FUNCTION "SEGNALAZIONI" : VOID
TITLE =SEGNALAZIONI
VERSION : 0.1

BEGIN
NETWORK
TITLE =SEGN 1 = TEMPERATURA MIN FORNO
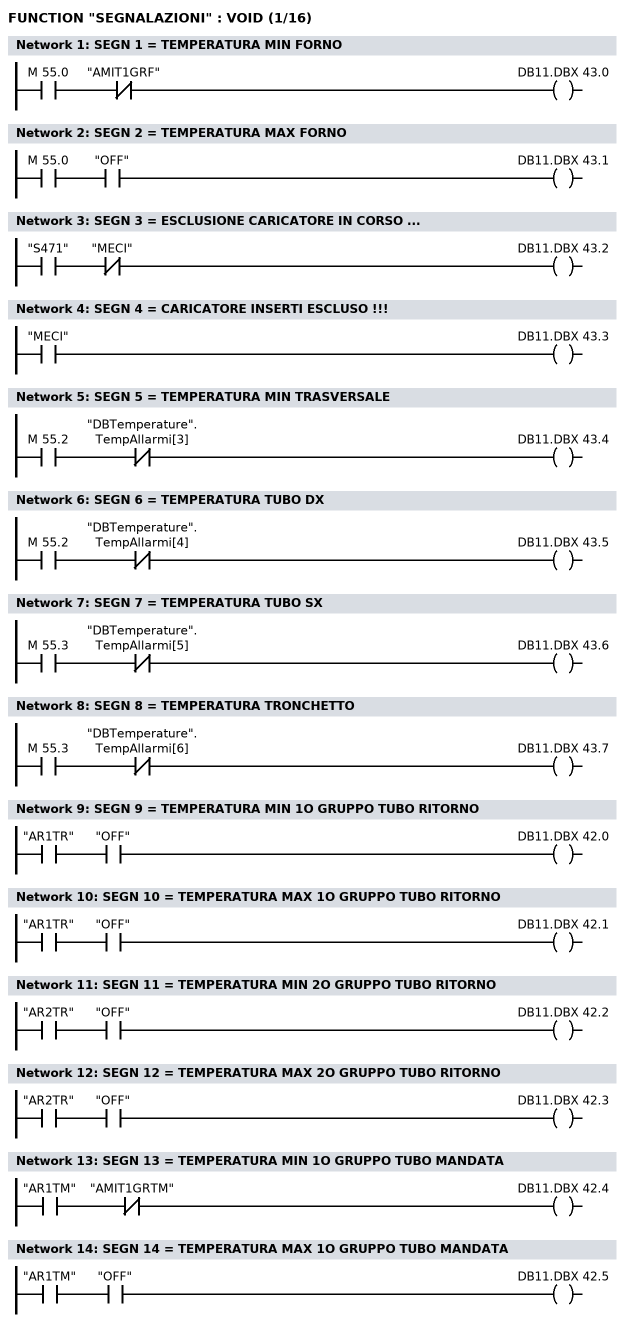
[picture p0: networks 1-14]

      U     M     55.0;
      UN    "AMIT1GRF";
      =     DB11.DBX   43.0;
NETWORK
TITLE =SEGN 2 = TEMPERATURA MAX FORNO

      U     M     55.0;
      U     "OFF";
      =     DB11.DBX   43.1;
NETWORK
TITLE =SEGN 3 = ESCLUSIONE CARICATORE IN CORSO ...

      U     "S471";
      UN    "MECI";
      =     DB11.DBX   43.2;
NETWORK
TITLE =SEGN 4 = CARICATORE INSERTI ESCLUSO !!!

      U     "MECI";
      =     DB11.DBX   43.3;
NETWORK
TITLE =SEGN 5 = TEMPERATURA MIN TRASVERSALE

      U     M     55.2;
      UN    "DBTemperature".TempAllarmi[3];
      =     DB11.DBX   43.4;
NETWORK
TITLE =SEGN 6 = TEMPERATURA TUBO DX

      U     M     55.2;
      UN    "DBTemperature".TempAllarmi[4];
      =     DB11.DBX   43.5;
NETWORK
TITLE =SEGN 7 = TEMPERATURA TUBO SX

      U     M     55.3;
      UN    "DBTemperature".TempAllarmi[5];
      =     DB11.DBX   43.6;
NETWORK
TITLE =SEGN 8 = TEMPERATURA TRONCHETTO

      U     M     55.3;
      UN    "DBTemperature".TempAllarmi[6];
      =     DB11.DBX   43.7;
NETWORK
TITLE =SEGN 9 = TEMPERATURA MIN 1O GRUPPO TUBO RITORNO

      U     "AR1TR";
      U     "OFF";
      =     DB11.DBX   42.0;
NETWORK
TITLE =SEGN 10 = TEMPERATURA MAX 1O GRUPPO TUBO RITORNO

      U     "AR1TR";
      U     "OFF";
      =     DB11.DBX   42.1;
NETWORK
TITLE =SEGN 11 = TEMPERATURA MIN 2O GRUPPO TUBO RITORNO

      U     "AR2TR";
      U     "OFF";
      =     DB11.DBX   42.2;
NETWORK
TITLE =SEGN 12 = TEMPERATURA MAX 2O GRUPPO TUBO RITORNO

      U     "AR2TR";
      U     "OFF";
      =     DB11.DBX   42.3;
NETWORK
TITLE =SEGN 13 = TEMPERATURA MIN 1O GRUPPO TUBO MANDATA

      U     "AR1TM";
      UN    "AMIT1GRTM";
      =     DB11.DBX   42.4;
NETWORK
TITLE =SEGN 14 = TEMPERATURA MAX 1O GRUPPO TUBO MANDATA

      U     "AR1TM";
      U     "OFF";
      =     DB11.DBX   42.5;
NETWORK
TITLE =SEGN 15 = TEMPERATURA MIN 2O GRUPPO TUBO MANDATA
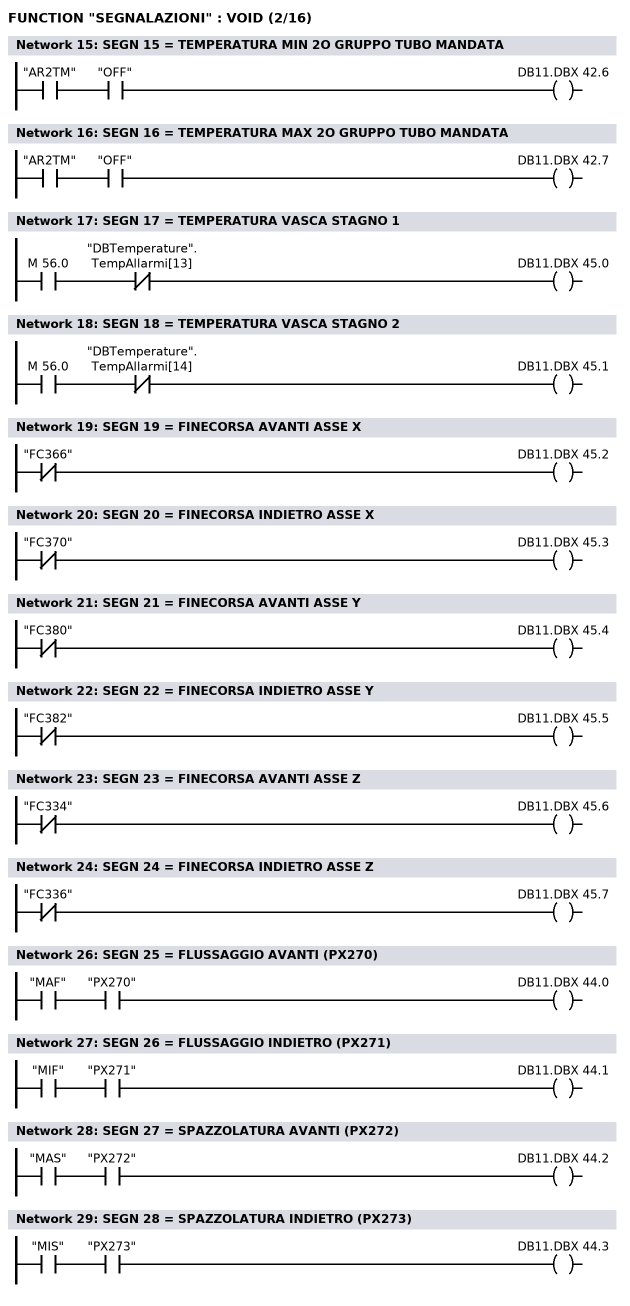
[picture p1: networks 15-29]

      U     "AR2TM";
      U     "OFF";
      =     DB11.DBX   42.6;
NETWORK
TITLE =SEGN 16 = TEMPERATURA MAX 2O GRUPPO TUBO MANDATA

      U     "AR2TM";
      U     "OFF";
      =     DB11.DBX   42.7;
NETWORK
TITLE =SEGN 17 = TEMPERATURA VASCA STAGNO 1

      U     M     56.0;
      UN    "DBTemperature".TempAllarmi[13];
      =     DB11.DBX   45.0;
NETWORK
TITLE =SEGN 18 = TEMPERATURA VASCA STAGNO 2

      U     M     56.0;
      UN    "DBTemperature".TempAllarmi[14];
      =     DB11.DBX   45.1;
NETWORK
TITLE =SEGN 19 = FINECORSA AVANTI ASSE X

      UN    "FC366";
      =     DB11.DBX   45.2;
NETWORK
TITLE =SEGN 20 = FINECORSA INDIETRO ASSE X

      UN    "FC370";
      =     DB11.DBX   45.3;
NETWORK
TITLE =SEGN 21 = FINECORSA AVANTI ASSE Y

      UN    "FC380";
      =     DB11.DBX   45.4;
NETWORK
TITLE =SEGN 22 = FINECORSA INDIETRO ASSE Y

      UN    "FC382";
      =     DB11.DBX   45.5;
NETWORK
TITLE =SEGN 23 = FINECORSA AVANTI ASSE Z

      UN    "FC334";
      =     DB11.DBX   45.6;
NETWORK
TITLE =SEGN 24 = FINECORSA INDIETRO ASSE Z

      UN    "FC336";
      =     DB11.DBX   45.7;
NETWORK
TITLE =

// ###########################################
// CONDIZIONI MOVIMENTI MANUALI
// ###########################################
NETWORK
TITLE =SEGN 25 = FLUSSAGGIO AVANTI (PX270)

      U     "MAF";
      U     "PX270";
      =     DB11.DBX   44.0;
NETWORK
TITLE =SEGN 26 = FLUSSAGGIO INDIETRO (PX271)

      U     "MIF";
      U     "PX271";
      =     DB11.DBX   44.1;
NETWORK
TITLE =SEGN 27 = SPAZZOLATURA AVANTI (PX272)

      U     "MAS";
      U     "PX272";
      =     DB11.DBX   44.2;
NETWORK
TITLE =SEGN 28 = SPAZZOLATURA INDIETRO (PX273)

      U     "MIS";
      U     "PX273";
      =     DB11.DBX   44.3;
NETWORK
TITLE =BIT TEST CONDIZIONI START ROTAZIONE
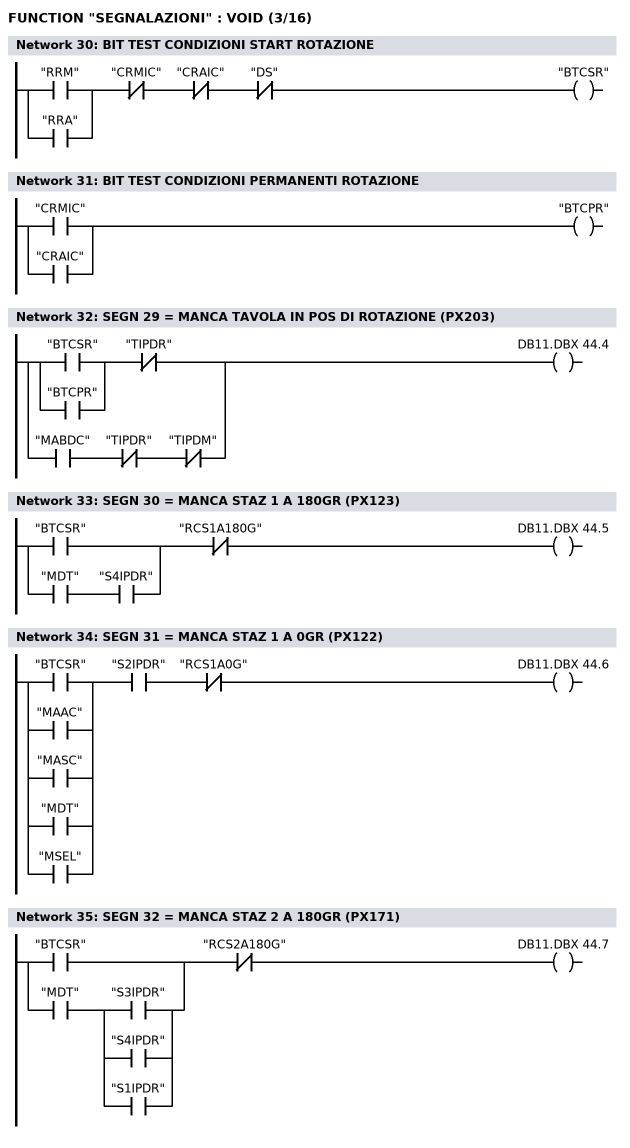
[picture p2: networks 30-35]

      U(    ;
      O     "RRM";
      O     "RRA";
      )     ;
      UN    "CRMIC";
      UN    "CRAIC";
      UN    "DS";
      =     "BTCSR";
NETWORK
TITLE =BIT TEST CONDIZIONI PERMANENTI ROTAZIONE

      O     "CRMIC";
      O     "CRAIC";
      =     "BTCPR";
NETWORK
TITLE =SEGN 29 = MANCA TAVOLA IN POS DI ROTAZIONE (PX203)

      U(    ;
      O     "BTCSR";
      O     "BTCPR";
      )     ;
      UN    "TIPDR";
      O     ;
      U     "MABDC";
      UN    "TIPDR";
      UN    "TIPDM";
      =     DB11.DBX   44.4;
NETWORK
TITLE =SEGN 30 = MANCA STAZ 1 A 180GR (PX123)

      U(    ;
      O     "BTCSR";
      O     ;
      U     "MDT";
      U     "S4IPDR";
      )     ;
      UN    "RCS1A180G";
      =     DB11.DBX   44.5;
NETWORK
TITLE =SEGN 31 = MANCA STAZ 1 A 0GR (PX122)

      U(    ;
      O     "BTCSR";
      O     "MAAC";
      O     "MASC";
      O     "MDT";
      O     "MSEL";
      )     ;
      U     "S2IPDR";
      UN    "RCS1A0G";
      =     DB11.DBX   44.6;
NETWORK
TITLE =SEGN 32 = MANCA STAZ 2 A 180GR (PX171)

      U(    ;
      O     "BTCSR";
      O     ;
      U     "MDT";
      U(    ;
      O     "S3IPDR";
      O     "S4IPDR";
      O     "S1IPDR";
      )     ;
      )     ;
      UN    "RCS2A180G";
      =     DB11.DBX   44.7;
NETWORK
TITLE =SEGN 33 = MANCA STAZ 2 A 0GR (PX170)
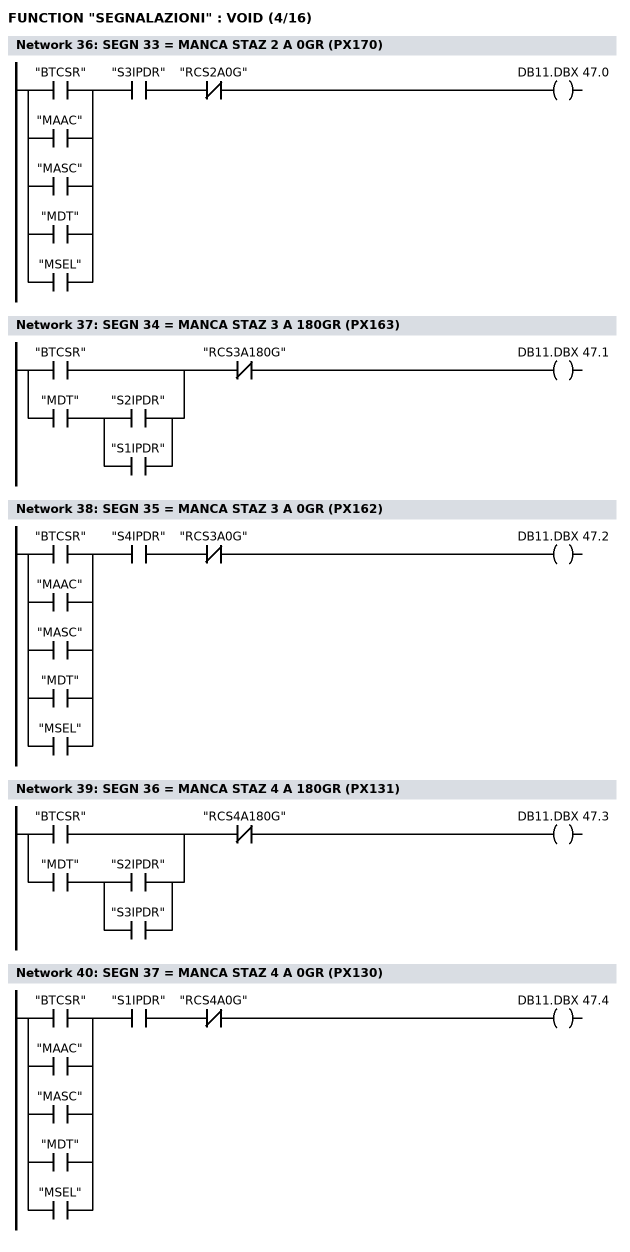
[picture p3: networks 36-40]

      U(    ;
      O     "BTCSR";
      O     "MAAC";
      O     "MASC";
      O     "MDT";
      O     "MSEL";
      )     ;
      U     "S3IPDR";
      UN    "RCS2A0G";
      =     DB11.DBX   47.0;
NETWORK
TITLE =SEGN 34 = MANCA STAZ 3 A 180GR (PX163)

      U(    ;
      O     "BTCSR";
      O     ;
      U     "MDT";
      U(    ;
      O     "S2IPDR";
      O     "S1IPDR";
      )     ;
      )     ;
      UN    "RCS3A180G";
      =     DB11.DBX   47.1;
NETWORK
TITLE =SEGN 35 = MANCA STAZ 3 A 0GR (PX162)

      U(    ;
      O     "BTCSR";
      O     "MAAC";
      O     "MASC";
      O     "MDT";
      O     "MSEL";
      )     ;
      U     "S4IPDR";
      UN    "RCS3A0G";
      =     DB11.DBX   47.2;
NETWORK
TITLE =SEGN 36 = MANCA STAZ 4 A 180GR (PX131)

      U(    ;
      O     "BTCSR";
      O     ;
      U     "MDT";
      U(    ;
      O     "S2IPDR";
      O     "S3IPDR";
      )     ;
      )     ;
      UN    "RCS4A180G";
      =     DB11.DBX   47.3;
NETWORK
TITLE =SEGN 37 = MANCA STAZ 4 A 0GR (PX130)

      U(    ;
      O     "BTCSR";
      O     "MAAC";
      O     "MASC";
      O     "MDT";
      O     "MSEL";
      )     ;
      U     "S1IPDR";
      UN    "RCS4A0G";
      =     DB11.DBX   47.4;
NETWORK
TITLE =SEGN 38 = MANCA BRACCIO DI CARICO INDIETRO (QUOTA)
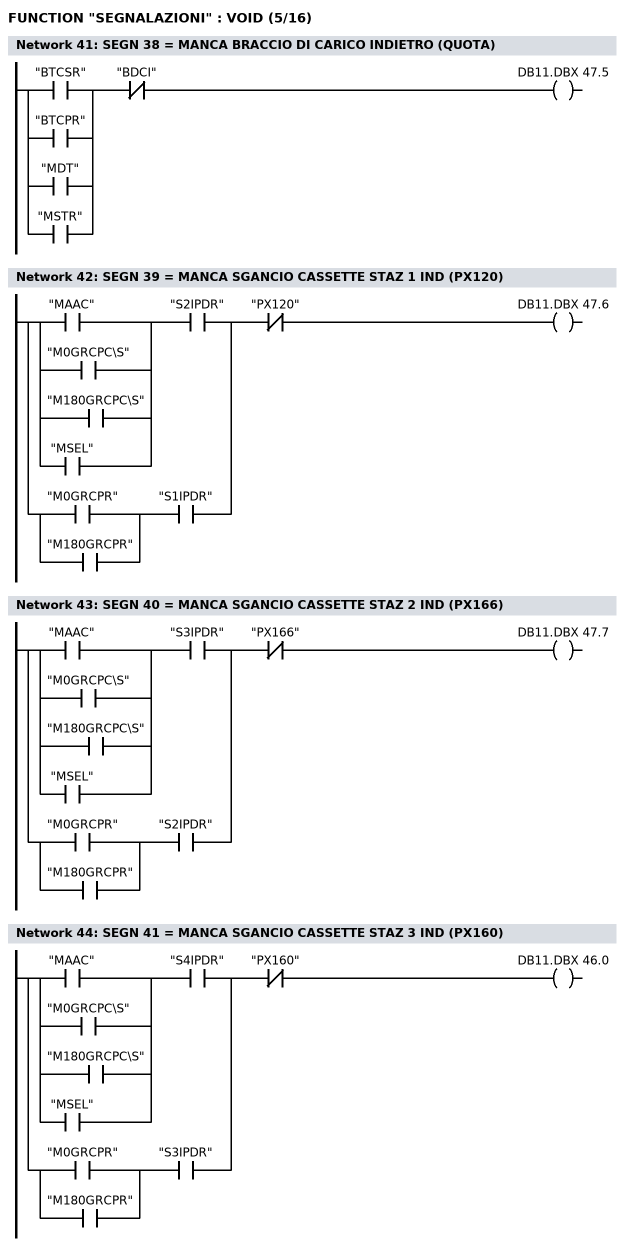
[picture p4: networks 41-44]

      U(    ;
      O     "BTCSR";
      O     "BTCPR";
      O     "MDT";
      O     "MSTR";
      )     ;
      UN    "BDCI";
      =     DB11.DBX   47.5;
NETWORK
TITLE =SEGN 39 = MANCA SGANCIO CASSETTE STAZ 1 IND (PX120)

      U(    ;
      U(    ;
      O     "MAAC";
      O     "M0GRCPC\S";
      O     "M180GRCPC\S";
      O     "MSEL";
      )     ;
      U     "S2IPDR";
      O     ;
      U(    ;
      O     "M0GRCPR";
      O     "M180GRCPR";
      )     ;
      U     "S1IPDR";
      )     ;
      UN    "PX120";
      =     DB11.DBX   47.6;
NETWORK
TITLE =SEGN 40 = MANCA SGANCIO CASSETTE STAZ 2 IND (PX166)

      U(    ;
      U(    ;
      O     "MAAC";
      O     "M0GRCPC\S";
      O     "M180GRCPC\S";
      O     "MSEL";
      )     ;
      U     "S3IPDR";
      O     ;
      U(    ;
      O     "M0GRCPR";
      O     "M180GRCPR";
      )     ;
      U     "S2IPDR";
      )     ;
      UN    "PX166";
      =     DB11.DBX   47.7;
NETWORK
TITLE =SEGN 41 = MANCA SGANCIO CASSETTE STAZ 3 IND (PX160)

      U(    ;
      U(    ;
      O     "MAAC";
      O     "M0GRCPC\S";
      O     "M180GRCPC\S";
      O     "MSEL";
      )     ;
      U     "S4IPDR";
      O     ;
      U(    ;
      O     "M0GRCPR";
      O     "M180GRCPR";
      )     ;
      U     "S3IPDR";
      )     ;
      UN    "PX160";
      =     DB11.DBX   46.0;
NETWORK
TITLE =SEGN 42 = MANCA SGANCIO CASSETTE STAZ 4 IND (PX126)
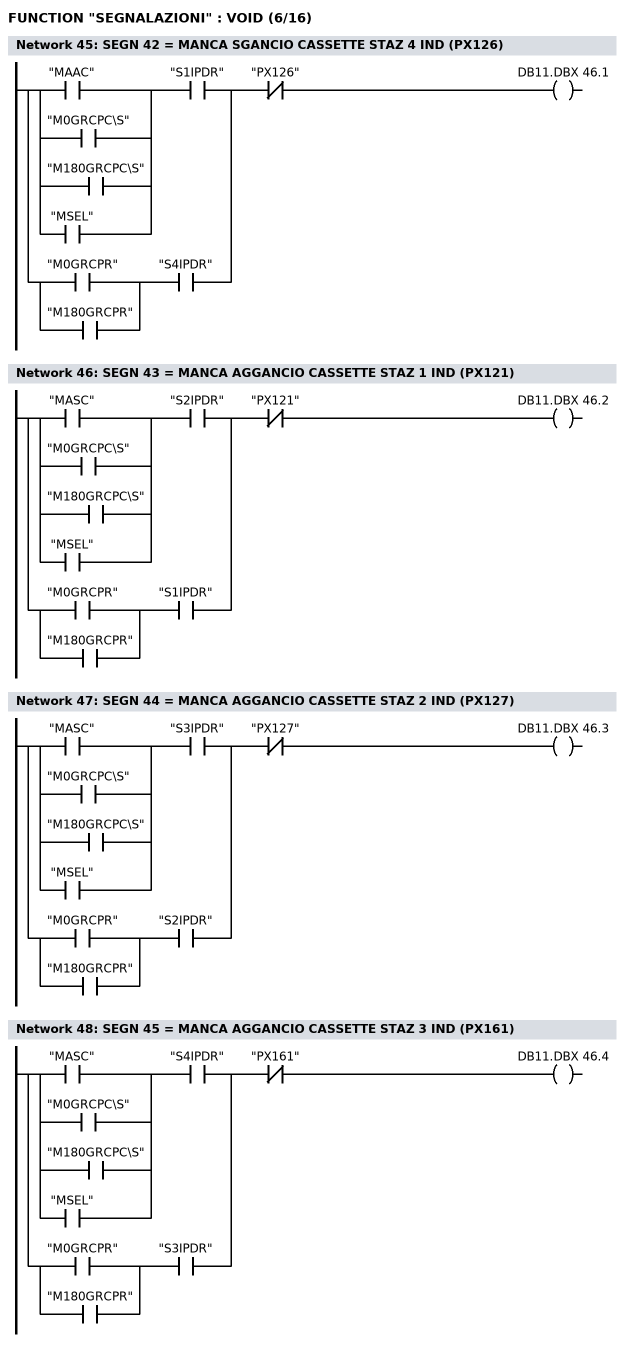
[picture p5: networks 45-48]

      U(    ;
      U(    ;
      O     "MAAC";
      O     "M0GRCPC\S";
      O     "M180GRCPC\S";
      O     "MSEL";
      )     ;
      U     "S1IPDR";
      O     ;
      U(    ;
      O     "M0GRCPR";
      O     "M180GRCPR";
      )     ;
      U     "S4IPDR";
      )     ;
      UN    "PX126";
      =     DB11.DBX   46.1;
NETWORK
TITLE =SEGN 43 = MANCA AGGANCIO CASSETTE STAZ 1 IND (PX121)

      U(    ;
      U(    ;
      O     "MASC";
      O     "M0GRCPC\S";
      O     "M180GRCPC\S";
      O     "MSEL";
      )     ;
      U     "S2IPDR";
      O     ;
      U(    ;
      O     "M0GRCPR";
      O     "M180GRCPR";
      )     ;
      U     "S1IPDR";
      )     ;
      UN    "PX121";
      =     DB11.DBX   46.2;
NETWORK
TITLE =SEGN 44 = MANCA AGGANCIO CASSETTE STAZ 2 IND (PX127)

      U(    ;
      U(    ;
      O     "MASC";
      O     "M0GRCPC\S";
      O     "M180GRCPC\S";
      O     "MSEL";
      )     ;
      U     "S3IPDR";
      O     ;
      U(    ;
      O     "M0GRCPR";
      O     "M180GRCPR";
      )     ;
      U     "S2IPDR";
      )     ;
      UN    "PX127";
      =     DB11.DBX   46.3;
NETWORK
TITLE =SEGN 45 = MANCA AGGANCIO CASSETTE STAZ 3 IND (PX161)

      U(    ;
      U(    ;
      O     "MASC";
      O     "M0GRCPC\S";
      O     "M180GRCPC\S";
      O     "MSEL";
      )     ;
      U     "S4IPDR";
      O     ;
      U(    ;
      O     "M0GRCPR";
      O     "M180GRCPR";
      )     ;
      U     "S3IPDR";
      )     ;
      UN    "PX161";
      =     DB11.DBX   46.4;
NETWORK
TITLE =SEGN 46 = MANCA AGGANCIO CASSETTE STAZ 4 IND (PX167)
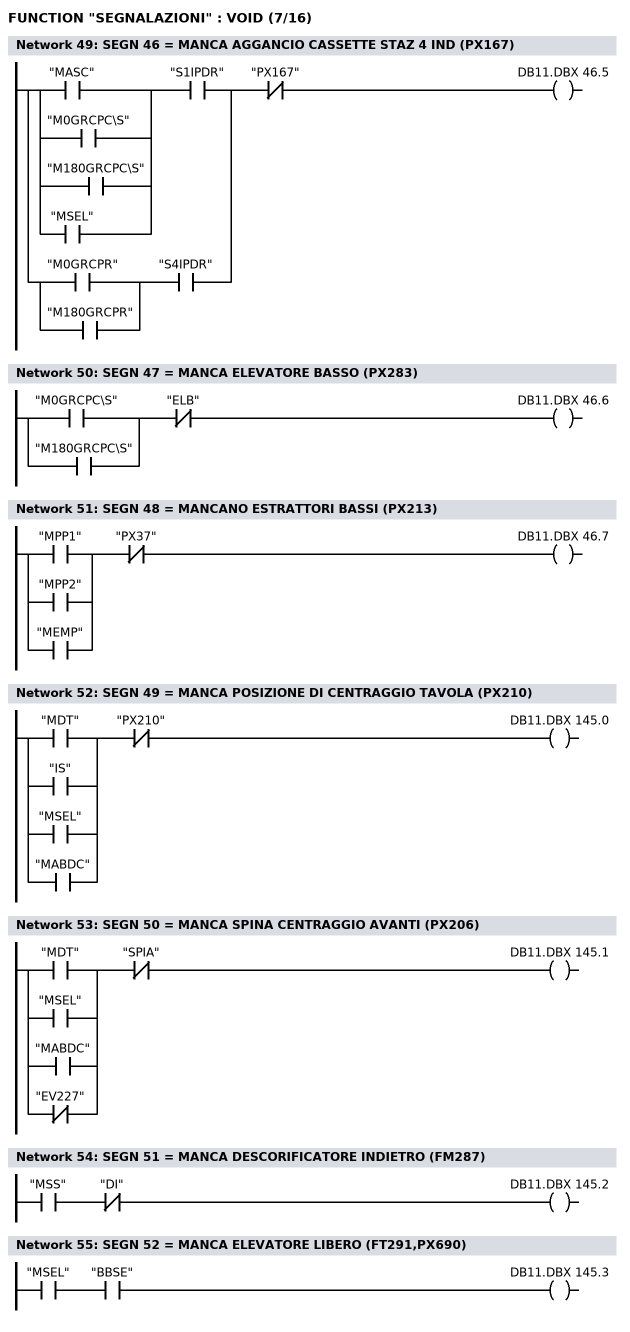
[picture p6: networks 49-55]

      U(    ;
      U(    ;
      O     "MASC";
      O     "M0GRCPC\S";
      O     "M180GRCPC\S";
      O     "MSEL";
      )     ;
      U     "S1IPDR";
      O     ;
      U(    ;
      O     "M0GRCPR";
      O     "M180GRCPR";
      )     ;
      U     "S4IPDR";
      )     ;
      UN    "PX167";
      =     DB11.DBX   46.5;
NETWORK
TITLE =SEGN 47 = MANCA ELEVATORE BASSO (PX283)

      U(    ;
      O     "M0GRCPC\S";
      O     "M180GRCPC\S";
      )     ;
      UN    "ELB";
      =     DB11.DBX   46.6;
NETWORK
TITLE =SEGN 48 = MANCANO ESTRATTORI BASSI (PX213)

      U(    ;
      O     "MPP1";
      O     "MPP2";
      O     "MEMP";
      )     ;
      UN    "PX37";
      =     DB11.DBX   46.7;
NETWORK
TITLE =SEGN 49 = MANCA POSIZIONE DI CENTRAGGIO TAVOLA (PX210)

      U(    ;
      O     "MDT";
      O     "IS";
      O     "MSEL";
      O     "MABDC";
      )     ;
      UN    "PX210";
      =     DB11.DBX  145.0;
NETWORK
TITLE =SEGN 50 = MANCA SPINA CENTRAGGIO AVANTI (PX206)

      U(    ;
      O     "MDT";
      O     "MSEL";
      O     "MABDC";
      ON    "EV227";
      )     ;
      UN    "SPIA";
      =     DB11.DBX  145.1;
NETWORK
TITLE =SEGN 51 = MANCA DESCORIFICATORE INDIETRO (FM287)

      U     "MSS";
      UN    "DI";
      =     DB11.DBX  145.2;
NETWORK
TITLE =SEGN 52 = MANCA ELEVATORE LIBERO (FT291,PX690)

      U     "MSEL";
      U     "BBSE";
      =     DB11.DBX  145.3;
NETWORK
TITLE =SEGN 53 = MANCA STAGNATURA BASSA (PX285)
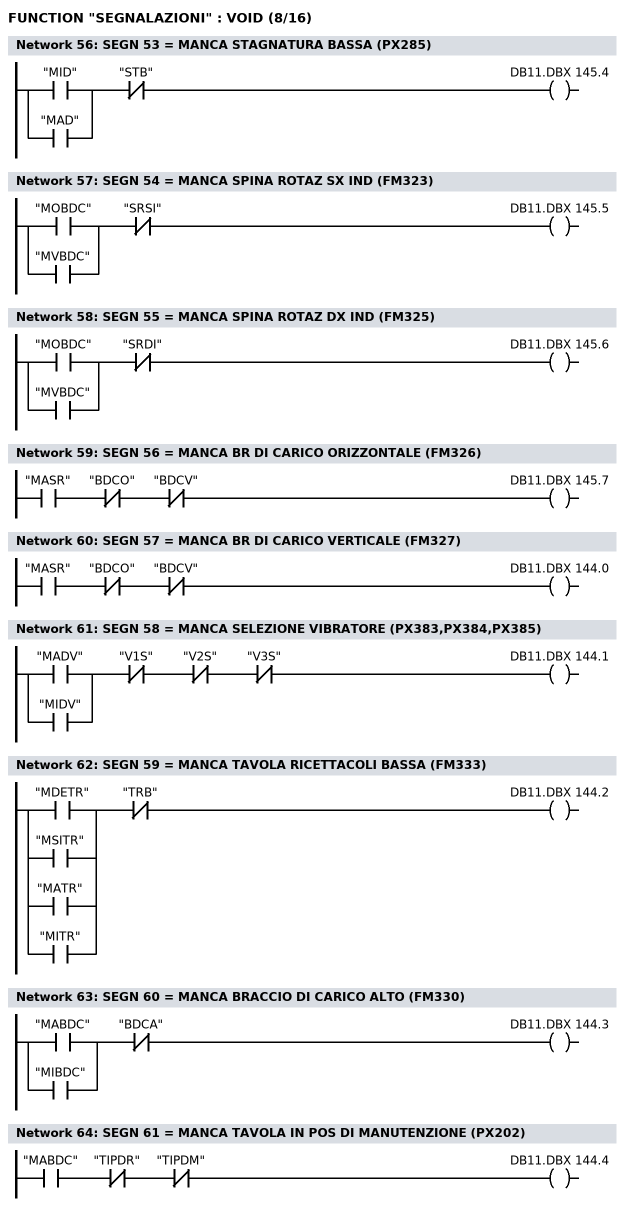
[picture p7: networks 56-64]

      U(    ;
      O     "MID";
      O     "MAD";
      )     ;
      UN    "STB";
      =     DB11.DBX  145.4;
NETWORK
TITLE =SEGN 54 = MANCA SPINA ROTAZ SX IND (FM323)

      U(    ;
      O     "MOBDC";
      O     "MVBDC";
      )     ;
      UN    "SRSI";
      =     DB11.DBX  145.5;
NETWORK
TITLE =SEGN 55 = MANCA SPINA ROTAZ DX IND (FM325)

      U(    ;
      O     "MOBDC";
      O     "MVBDC";
      )     ;
      UN    "SRDI";
      =     DB11.DBX  145.6;
NETWORK
TITLE =SEGN 56 = MANCA BR DI CARICO ORIZZONTALE (FM326)

      U     "MASR";
      UN    "BDCO";
      UN    "BDCV";
      =     DB11.DBX  145.7;
NETWORK
TITLE =SEGN 57 = MANCA BR DI CARICO VERTICALE (FM327)

      U     "MASR";
      UN    "BDCO";
      UN    "BDCV";
      =     DB11.DBX  144.0;
NETWORK
TITLE =SEGN 58 = MANCA SELEZIONE VIBRATORE (PX383,PX384,PX385)

      U(    ;
      O     "MADV";
      O     "MIDV";
      )     ;
      UN    "V1S";
      UN    "V2S";
      UN    "V3S";
      =     DB11.DBX  144.1;
NETWORK
TITLE =SEGN 59 = MANCA TAVOLA RICETTACOLI BASSA (FM333)

      U(    ;
      O     "MDETR";
      O     "MSITR";
      O     "MATR";
      O     "MITR";
      )     ;
      UN    "TRB";
      =     DB11.DBX  144.2;
NETWORK
TITLE =SEGN 60 = MANCA BRACCIO DI CARICO ALTO (FM330)

      U(    ;
      O     "MABDC";
      O     "MIBDC";
      )     ;
      UN    "BDCA";
      =     DB11.DBX  144.3;
NETWORK
TITLE =SEGN 61 = MANCA TAVOLA IN POS DI MANUTENZIONE (PX202)

      U     "MABDC";
      UN    "TIPDR";
      UN    "TIPDM";
      =     DB11.DBX  144.4;
NETWORK
TITLE =SEGN 62 = MANCA POSIZIONE STAZIONI (PX114,PX115,PX116,PX117)
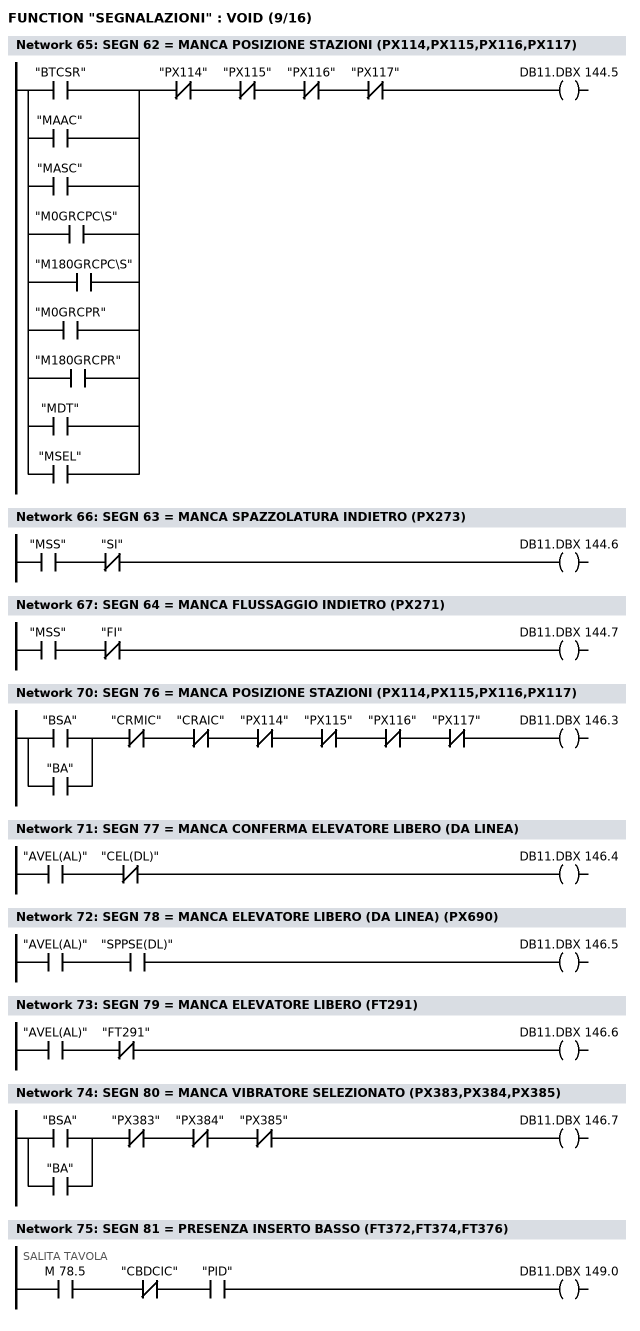
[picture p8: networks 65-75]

      U(    ;
      O     "BTCSR";
      O     "MAAC";
      O     "MASC";
      O     "M0GRCPC\S";
      O     "M180GRCPC\S";
      O     "M0GRCPR";
      O     "M180GRCPR";
      O     "MDT";
      O     "MSEL";
      )     ;
      UN    "PX114";
      UN    "PX115";
      UN    "PX116";
      UN    "PX117";
      =     DB11.DBX  144.5;
NETWORK
TITLE =SEGN 63 = MANCA SPAZZOLATURA INDIETRO (PX273)

      U     "MSS";
      UN    "SI";
      =     DB11.DBX  144.6;
NETWORK
TITLE =SEGN 64 = MANCA FLUSSAGGIO INDIETRO (PX271)

      U     "MSS";
      UN    "FI";
      =     DB11.DBX  144.7;
NETWORK
TITLE =

// SEGN 65-72 DBB147
// SEGN 73-80 DBB146
NETWORK
TITLE =

// ###########################################
// CONTROLLO SEGNALI SENZA COMANDO
// ###########################################
NETWORK
TITLE =SEGN 76 = MANCA POSIZIONE STAZIONI (PX114,PX115,PX116,PX117)

      U(    ;
      O     "BSA";
      O     "BA";
      )     ;
      UN    "CRMIC";
      UN    "CRAIC";
      UN    "PX114";
      UN    "PX115";
      UN    "PX116";
      UN    "PX117";
      =     DB11.DBX  146.3;
NETWORK
TITLE =SEGN 77 = MANCA CONFERMA ELEVATORE LIBERO (DA LINEA)

      U     "AVEL(AL)";
      UN    "CEL(DL)";
      =     DB11.DBX  146.4;
NETWORK
TITLE =SEGN 78 = MANCA ELEVATORE LIBERO (DA LINEA) (PX690)

      U     "AVEL(AL)";
      U     "SPPSE(DL)";
      =     DB11.DBX  146.5;
NETWORK
TITLE =SEGN 79 = MANCA ELEVATORE LIBERO (FT291)

      U     "AVEL(AL)";
      UN    "FT291";
      =     DB11.DBX  146.6;
NETWORK
TITLE =SEGN 80 = MANCA VIBRATORE SELEZIONATO (PX383,PX384,PX385)

      U(    ;
      O     "BSA";
      O     "BA";
      )     ;
      UN    "PX383";
      UN    "PX384";
      UN    "PX385";
      =     DB11.DBX  146.7;
NETWORK
TITLE =SEGN 81 = PRESENZA INSERTO BASSO (FT372,FT374,FT376)

      U     M     78.5; // SALITA TAVOLA
      UN    "CBDCIC";
      U     "PID";
      =     DB11.DBX  149.0;
NETWORK
TITLE =SEGN 82 = MANCA BRACCIO DI CARICO ALTO (FM330)
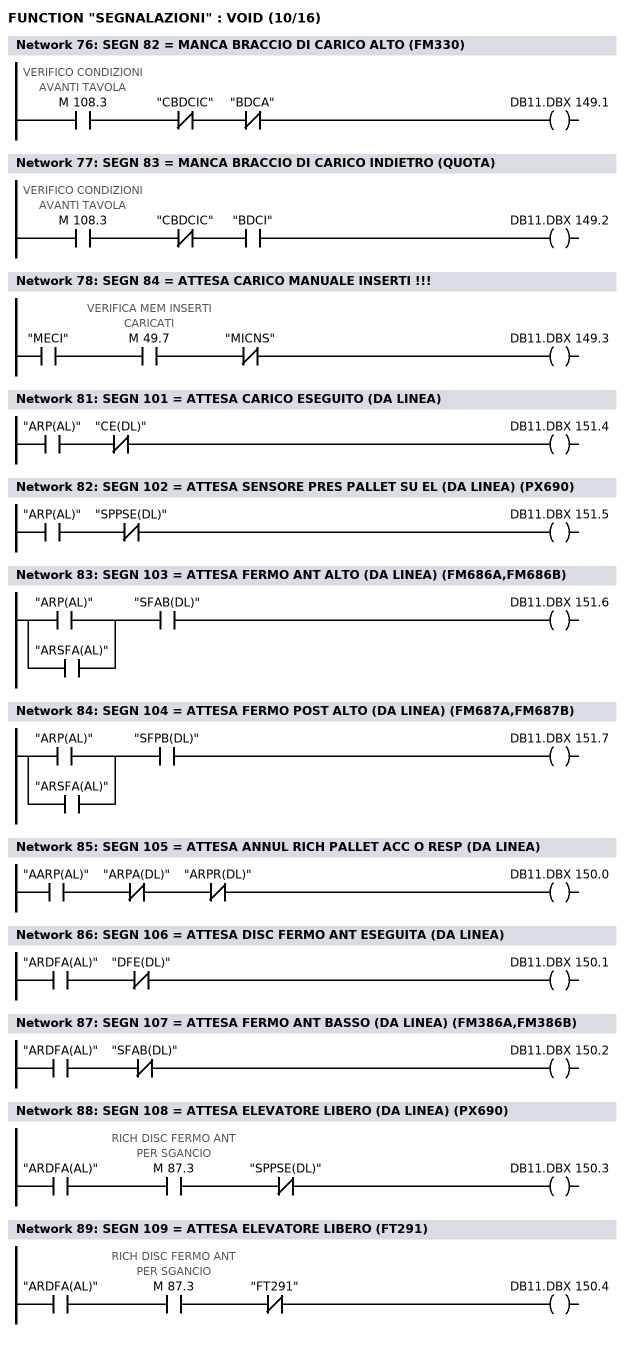
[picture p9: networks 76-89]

      U     M    108.3; // VERIFICO CONDIZIONI AVANTI TAVOLA
      UN    "CBDCIC";
      UN    "BDCA";
      =     DB11.DBX  149.1;
NETWORK
TITLE =SEGN 83 = MANCA BRACCIO DI CARICO INDIETRO (QUOTA)

      U     M    108.3; // VERIFICO CONDIZIONI AVANTI TAVOLA
      UN    "CBDCIC";
      U     "BDCI";
      =     DB11.DBX  149.2;
NETWORK
TITLE =SEGN 84 = ATTESA CARICO MANUALE INSERTI !!!

      U     "MECI";
      U     M     49.7; // VERIFICA MEM INSERTI CARICATI
      UN    "MICNS";
      =     DB11.DBX  149.3;
NETWORK
TITLE =

// SEGN 81-88 DBB149
// SEGN 89-96 DBB148
// SEGN 97-104 DBB151
NETWORK
TITLE =

// ###########################################
// CONTROLLO SEGNALI CON COMANDO
// ###########################################
NETWORK
TITLE =SEGN 101 = ATTESA CARICO ESEGUITO (DA LINEA)

      U     "ARP(AL)";
      UN    "CE(DL)";
      =     DB11.DBX  151.4;
NETWORK
TITLE =SEGN 102 = ATTESA SENSORE PRES PALLET SU EL (DA LINEA) (PX690)

      U     "ARP(AL)";
      UN    "SPPSE(DL)";
      =     DB11.DBX  151.5;
NETWORK
TITLE =SEGN 103 = ATTESA FERMO ANT ALTO (DA LINEA) (FM686A,FM686B)

      U(    ;
      O     "ARP(AL)";
      O     "ARSFA(AL)";
      )     ;
      U     "SFAB(DL)";
      =     DB11.DBX  151.6;
NETWORK
TITLE =SEGN 104 = ATTESA FERMO POST ALTO (DA LINEA) (FM687A,FM687B)

      U(    ;
      O     "ARP(AL)";
      O     "ARSFA(AL)";
      )     ;
      U     "SFPB(DL)";
      =     DB11.DBX  151.7;
NETWORK
TITLE =SEGN 105 = ATTESA ANNUL RICH PALLET ACC O RESP (DA LINEA)

      U     "AARP(AL)";
      UN    "ARPA(DL)";
      UN    "ARPR(DL)";
      =     DB11.DBX  150.0;
NETWORK
TITLE =SEGN 106 = ATTESA DISC FERMO ANT ESEGUITA (DA LINEA)

      U     "ARDFA(AL)";
      UN    "DFE(DL)";
      =     DB11.DBX  150.1;
NETWORK
TITLE =SEGN 107 = ATTESA FERMO ANT BASSO (DA LINEA) (FM386A,FM386B)

      U     "ARDFA(AL)";
      UN    "SFAB(DL)";
      =     DB11.DBX  150.2;
NETWORK
TITLE =SEGN 108 = ATTESA ELEVATORE LIBERO (DA LINEA) (PX690)

      U     "ARDFA(AL)";
      U     M     87.3; // RICH DISC FERMO ANT PER SGANCIO
      UN    "SPPSE(DL)";
      =     DB11.DBX  150.3;
NETWORK
TITLE =SEGN 109 = ATTESA ELEVATORE LIBERO (FT291)

      U     "ARDFA(AL)";
      U     M     87.3; // RICH DISC FERMO ANT PER SGANCIO
      UN    "FT291";
      =     DB11.DBX  150.4;
NETWORK
TITLE =SEGN 110 = ATTESA FERMO POST ALTO (DA LINEA) (FM387A,FM387B)
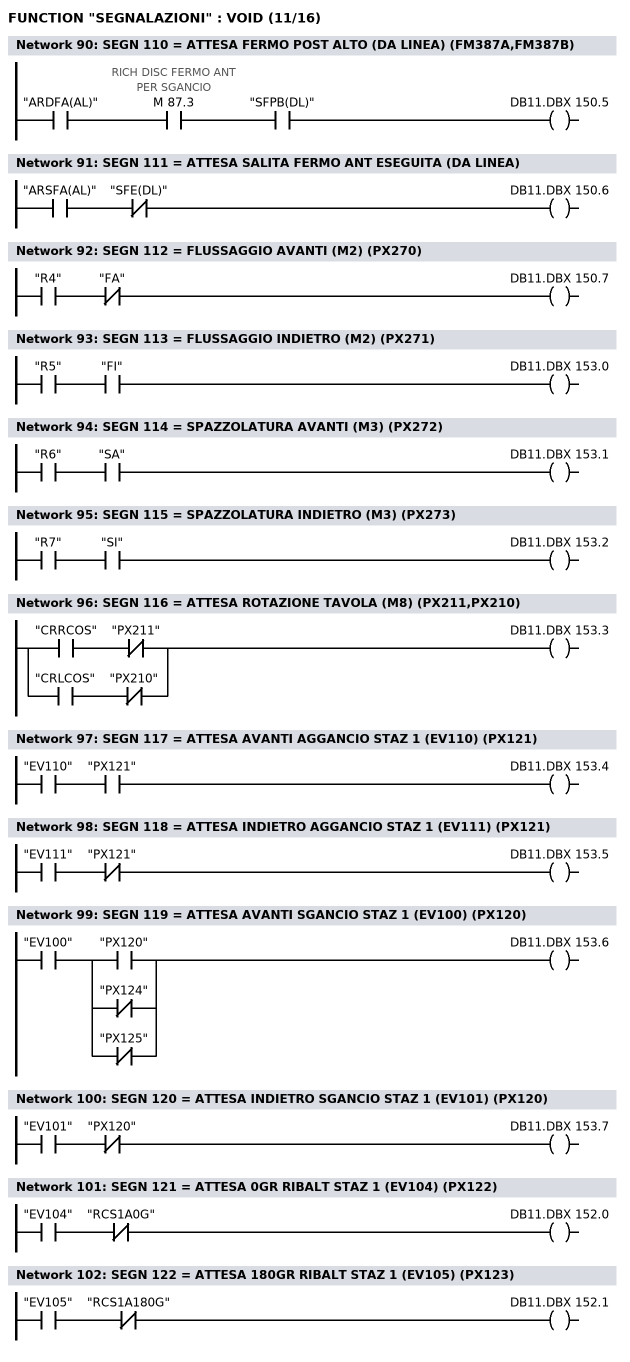
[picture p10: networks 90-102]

      U     "ARDFA(AL)";
      U     M     87.3; // RICH DISC FERMO ANT PER SGANCIO
      U     "SFPB(DL)";
      =     DB11.DBX  150.5;
NETWORK
TITLE =SEGN 111 = ATTESA SALITA FERMO ANT ESEGUITA (DA LINEA)

      U     "ARSFA(AL)";
      UN    "SFE(DL)";
      =     DB11.DBX  150.6;
NETWORK
TITLE =SEGN 112 = FLUSSAGGIO AVANTI (M2) (PX270)

      U     "R4";
      UN    "FA";
      =     DB11.DBX  150.7;
NETWORK
TITLE =SEGN 113 = FLUSSAGGIO INDIETRO (M2) (PX271)

      U     "R5";
      U     "FI";
      =     DB11.DBX  153.0;
NETWORK
TITLE =SEGN 114 = SPAZZOLATURA AVANTI (M3) (PX272)

      U     "R6";
      U     "SA";
      =     DB11.DBX  153.1;
NETWORK
TITLE =SEGN 115 = SPAZZOLATURA INDIETRO (M3) (PX273)

      U     "R7";
      U     "SI";
      =     DB11.DBX  153.2;
NETWORK
TITLE =SEGN 116 = ATTESA ROTAZIONE TAVOLA (M8) (PX211,PX210)

      U     "CRRCOS";
      UN    "PX211";
      O     ;
      U     "CRLCOS";
      UN    "PX210";
      =     DB11.DBX  153.3;
NETWORK
TITLE =SEGN 117 = ATTESA AVANTI AGGANCIO STAZ 1 (EV110) (PX121)

      U     "EV110";
      U     "PX121";
      =     DB11.DBX  153.4;
NETWORK
TITLE =SEGN 118 = ATTESA INDIETRO AGGANCIO STAZ 1 (EV111) (PX121)

      U     "EV111";
      UN    "PX121";
      =     DB11.DBX  153.5;
NETWORK
TITLE =SEGN 119 = ATTESA AVANTI SGANCIO STAZ 1 (EV100) (PX120)

      U     "EV100";
      U(    ;
      O     "PX120";
      ON    "PX124";
      ON    "PX125";
      )     ;
      =     DB11.DBX  153.6;
NETWORK
TITLE =SEGN 120 = ATTESA INDIETRO SGANCIO STAZ 1 (EV101) (PX120)

      U     "EV101";
      UN    "PX120";
      =     DB11.DBX  153.7;
NETWORK
TITLE =SEGN 121 = ATTESA 0GR RIBALT STAZ 1 (EV104) (PX122)

      U     "EV104";
      UN    "RCS1A0G";
      =     DB11.DBX  152.0;
NETWORK
TITLE =SEGN 122 = ATTESA 180GR RIBALT STAZ 1 (EV105) (PX123)

      U     "EV105";
      UN    "RCS1A180G";
      =     DB11.DBX  152.1;
NETWORK
TITLE =SEGN 123 = ATTESA AVANTI AGGANCIO STAZ 2 (EV102) (PX127)
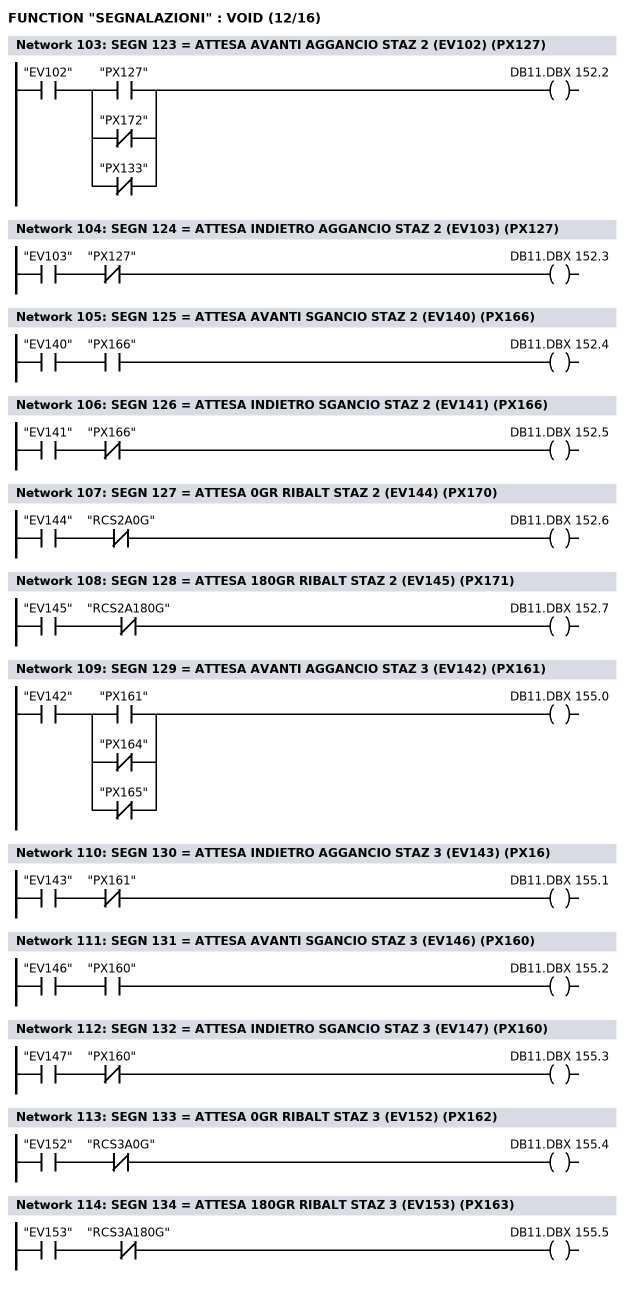
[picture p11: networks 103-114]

      U     "EV102";
      U(    ;
      O     "PX127";
      ON    "PX172";
      ON    "PX133";
      )     ;
      =     DB11.DBX  152.2;
NETWORK
TITLE =SEGN 124 = ATTESA INDIETRO AGGANCIO STAZ 2 (EV103) (PX127)

      U     "EV103";
      UN    "PX127";
      =     DB11.DBX  152.3;
NETWORK
TITLE =SEGN 125 = ATTESA AVANTI SGANCIO STAZ 2 (EV140) (PX166)

      U     "EV140";
      U     "PX166";
      =     DB11.DBX  152.4;
NETWORK
TITLE =SEGN 126 = ATTESA INDIETRO SGANCIO STAZ 2 (EV141) (PX166)

      U     "EV141";
      UN    "PX166";
      =     DB11.DBX  152.5;
NETWORK
TITLE =SEGN 127 = ATTESA 0GR RIBALT STAZ 2 (EV144) (PX170)

      U     "EV144";
      UN    "RCS2A0G";
      =     DB11.DBX  152.6;
NETWORK
TITLE =SEGN 128 = ATTESA 180GR RIBALT STAZ 2 (EV145) (PX171)

      U     "EV145";
      UN    "RCS2A180G";
      =     DB11.DBX  152.7;
NETWORK
TITLE =SEGN 129 = ATTESA AVANTI AGGANCIO STAZ 3 (EV142) (PX161)

      U     "EV142";
      U(    ;
      O     "PX161";
      ON    "PX164";
      ON    "PX165";
      )     ;
      =     DB11.DBX  155.0;
NETWORK
TITLE =SEGN 130 = ATTESA INDIETRO AGGANCIO STAZ 3 (EV143) (PX16)

      U     "EV143";
      UN    "PX161";
      =     DB11.DBX  155.1;
NETWORK
TITLE =SEGN 131 = ATTESA AVANTI SGANCIO STAZ 3 (EV146) (PX160)

      U     "EV146";
      U     "PX160";
      =     DB11.DBX  155.2;
NETWORK
TITLE =SEGN 132 = ATTESA INDIETRO SGANCIO STAZ 3 (EV147) (PX160)

      U     "EV147";
      UN    "PX160";
      =     DB11.DBX  155.3;
NETWORK
TITLE =SEGN 133 = ATTESA 0GR RIBALT STAZ 3 (EV152) (PX162)

      U     "EV152";
      UN    "RCS3A0G";
      =     DB11.DBX  155.4;
NETWORK
TITLE =SEGN 134 = ATTESA 180GR RIBALT STAZ 3 (EV153) (PX163)

      U     "EV153";
      UN    "RCS3A180G";
      =     DB11.DBX  155.5;
NETWORK
TITLE =SEGN 135 = ATTESA AVANTI AGGANCIO STAZ 4 (EV150) (PX167)
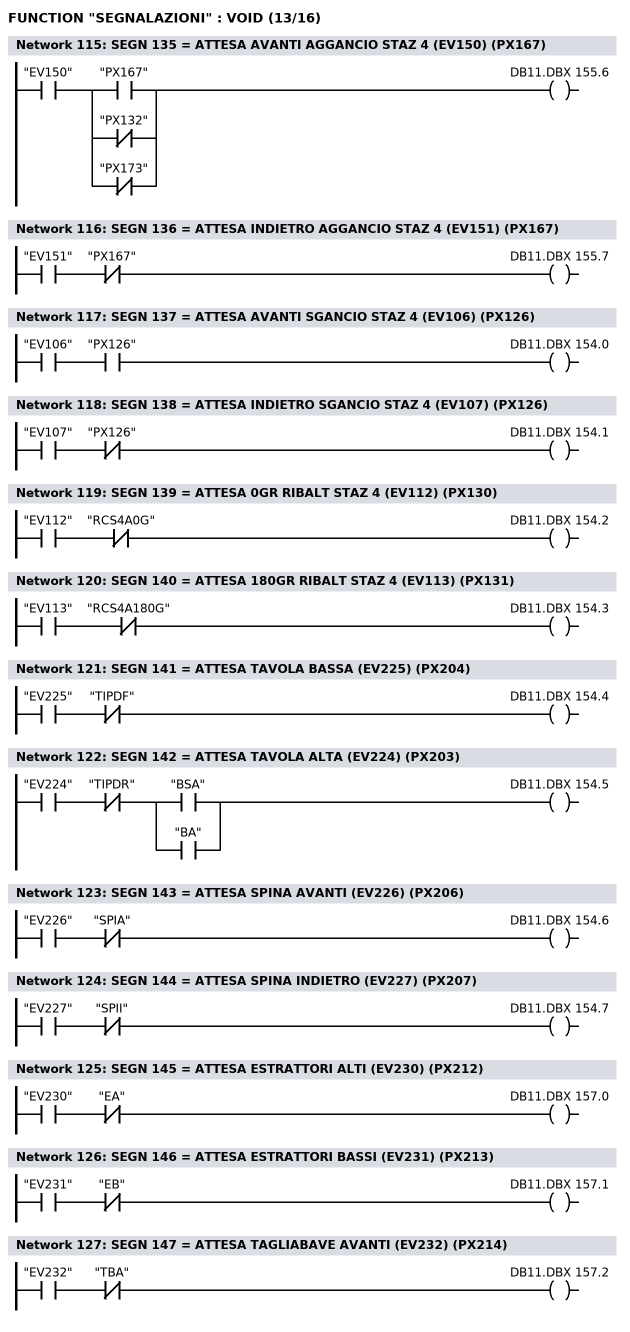
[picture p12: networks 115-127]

      U     "EV150";
      U(    ;
      O     "PX167";
      ON    "PX132";
      ON    "PX173";
      )     ;
      =     DB11.DBX  155.6;
NETWORK
TITLE =SEGN 136 = ATTESA INDIETRO AGGANCIO STAZ 4 (EV151) (PX167)

      U     "EV151";
      UN    "PX167";
      =     DB11.DBX  155.7;
NETWORK
TITLE =SEGN 137 = ATTESA AVANTI SGANCIO STAZ 4 (EV106) (PX126)

      U     "EV106";
      U     "PX126";
      =     DB11.DBX  154.0;
NETWORK
TITLE =SEGN 138 = ATTESA INDIETRO SGANCIO STAZ 4 (EV107) (PX126)

      U     "EV107";
      UN    "PX126";
      =     DB11.DBX  154.1;
NETWORK
TITLE =SEGN 139 = ATTESA 0GR RIBALT STAZ 4 (EV112) (PX130)

      U     "EV112";
      UN    "RCS4A0G";
      =     DB11.DBX  154.2;
NETWORK
TITLE =SEGN 140 = ATTESA 180GR RIBALT STAZ 4 (EV113) (PX131)

      U     "EV113";
      UN    "RCS4A180G";
      =     DB11.DBX  154.3;
NETWORK
TITLE =SEGN 141 = ATTESA TAVOLA BASSA (EV225) (PX204)

      U     "EV225";
      UN    "TIPDF";
      =     DB11.DBX  154.4;
NETWORK
TITLE =SEGN 142 = ATTESA TAVOLA ALTA (EV224) (PX203)

      U     "EV224";
      UN    "TIPDR";
      U(    ;
      O     "BSA";
      O     "BA";
      )     ;
      =     DB11.DBX  154.5;
NETWORK
TITLE =SEGN 143 = ATTESA SPINA AVANTI (EV226) (PX206)

      U     "EV226";
      UN    "SPIA";
      =     DB11.DBX  154.6;
NETWORK
TITLE =SEGN 144 = ATTESA SPINA INDIETRO (EV227) (PX207)

      U     "EV227";
      UN    "SPII";
      =     DB11.DBX  154.7;
NETWORK
TITLE =SEGN 145 = ATTESA ESTRATTORI ALTI (EV230) (PX212)

      U     "EV230";
      UN    "EA";
      =     DB11.DBX  157.0;
NETWORK
TITLE =SEGN 146 = ATTESA ESTRATTORI BASSI (EV231) (PX213)

      U     "EV231";
      UN    "EB";
      =     DB11.DBX  157.1;
NETWORK
TITLE =SEGN 147 = ATTESA TAGLIABAVE AVANTI (EV232) (PX214)

      U     "EV232";
      UN    "TBA";
      =     DB11.DBX  157.2;
NETWORK
TITLE =SEGN 148 = ATTESA TAGLIABAVE INDIETRO (EV233) (PX215)
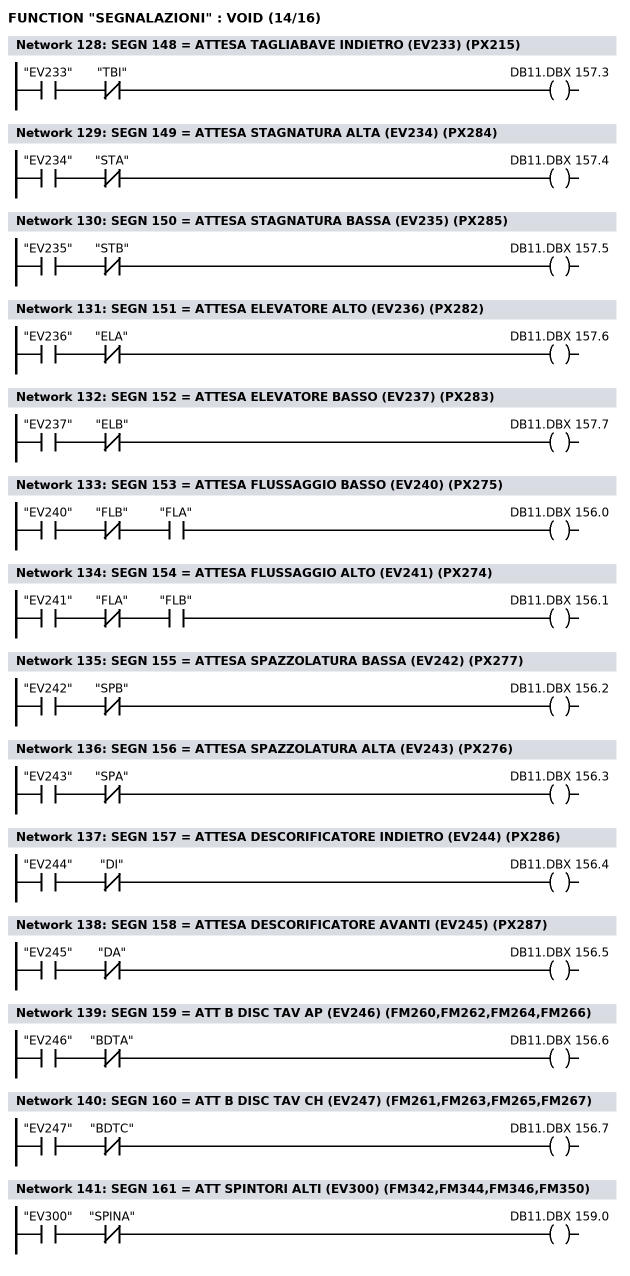
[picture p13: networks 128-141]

      U     "EV233";
      UN    "TBI";
      =     DB11.DBX  157.3;
NETWORK
TITLE =SEGN 149 = ATTESA STAGNATURA ALTA (EV234) (PX284)

      U     "EV234";
      UN    "STA";
      =     DB11.DBX  157.4;
NETWORK
TITLE =SEGN 150 = ATTESA STAGNATURA BASSA (EV235) (PX285)

      U     "EV235";
      UN    "STB";
      =     DB11.DBX  157.5;
NETWORK
TITLE =SEGN 151 = ATTESA ELEVATORE ALTO (EV236) (PX282)

      U     "EV236";
      UN    "ELA";
      =     DB11.DBX  157.6;
NETWORK
TITLE =SEGN 152 = ATTESA ELEVATORE BASSO (EV237) (PX283)

      U     "EV237";
      UN    "ELB";
      =     DB11.DBX  157.7;
NETWORK
TITLE =SEGN 153 = ATTESA FLUSSAGGIO BASSO (EV240) (PX275)

      U     "EV240";
      UN    "FLB";
      U     "FLA";
      =     DB11.DBX  156.0;
NETWORK
TITLE =SEGN 154 = ATTESA FLUSSAGGIO ALTO (EV241) (PX274)

      U     "EV241";
      UN    "FLA";
      U     "FLB";
      =     DB11.DBX  156.1;
NETWORK
TITLE =SEGN 155 = ATTESA SPAZZOLATURA BASSA (EV242) (PX277)

      U     "EV242";
      UN    "SPB";
      =     DB11.DBX  156.2;
NETWORK
TITLE =SEGN 156 = ATTESA SPAZZOLATURA ALTA (EV243) (PX276)

      U     "EV243";
      UN    "SPA";
      =     DB11.DBX  156.3;
NETWORK
TITLE =SEGN 157 = ATTESA DESCORIFICATORE INDIETRO (EV244) (PX286)

      U     "EV244";
      UN    "DI";
      =     DB11.DBX  156.4;
NETWORK
TITLE =SEGN 158 = ATTESA DESCORIFICATORE AVANTI (EV245) (PX287)

      U     "EV245";
      UN    "DA";
      =     DB11.DBX  156.5;
NETWORK
TITLE =SEGN 159 = ATT B DISC TAV AP (EV246) (FM260,FM262,FM264,FM266)

      U     "EV246";
      UN    "BDTA";
      =     DB11.DBX  156.6;
NETWORK
TITLE =SEGN 160 = ATT B DISC TAV CH (EV247) (FM261,FM263,FM265,FM267)

      U     "EV247";
      UN    "BDTC";
      =     DB11.DBX  156.7;
NETWORK
TITLE =SEGN 161 = ATT SPINTORI ALTI (EV300) (FM342,FM344,FM346,FM350)

      U     "EV300";
      UN    "SPINA";
      =     DB11.DBX  159.0;
NETWORK
TITLE =SEGN 162 = ATT SPINTORI BASSI (EV301) (FM343,FM345,FM347,FM351)
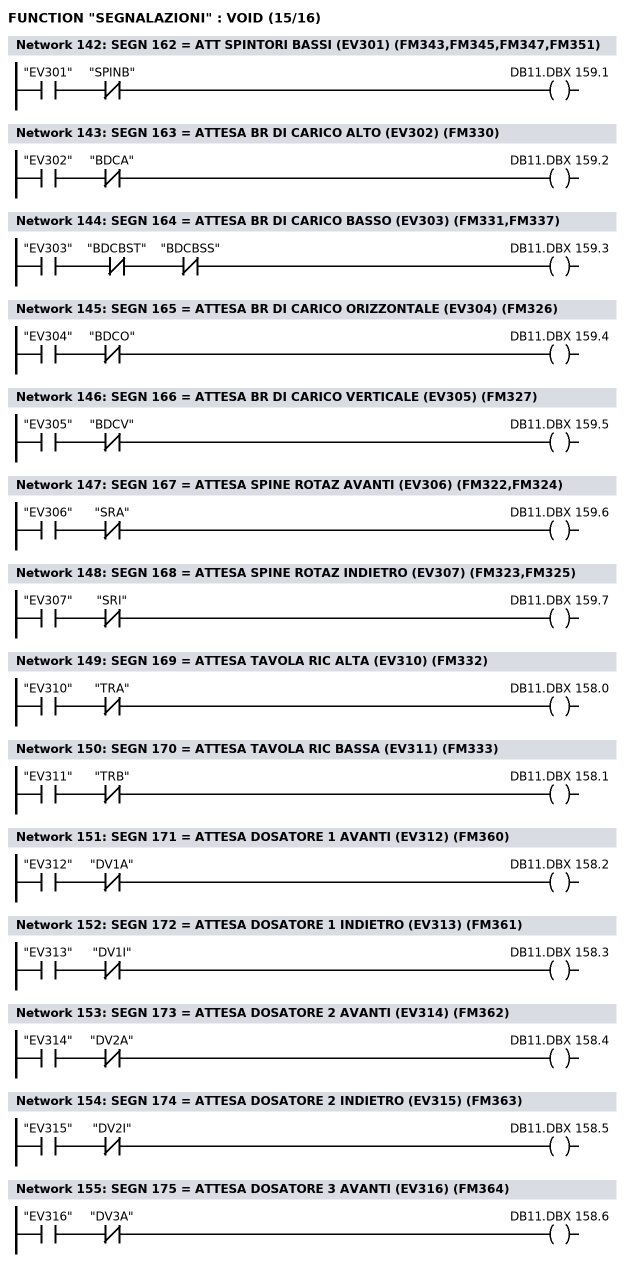
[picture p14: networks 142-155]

      U     "EV301";
      UN    "SPINB";
      =     DB11.DBX  159.1;
NETWORK
TITLE =SEGN 163 = ATTESA BR DI CARICO ALTO (EV302) (FM330)

      U     "EV302";
      UN    "BDCA";
      =     DB11.DBX  159.2;
NETWORK
TITLE =SEGN 164 = ATTESA BR DI CARICO BASSO (EV303) (FM331,FM337)

      U     "EV303";
      UN    "BDCBST";
      UN    "BDCBSS";
      =     DB11.DBX  159.3;
NETWORK
TITLE =SEGN 165 = ATTESA BR DI CARICO ORIZZONTALE (EV304) (FM326)

      U     "EV304";
      UN    "BDCO";
      =     DB11.DBX  159.4;
NETWORK
TITLE =SEGN 166 = ATTESA BR DI CARICO VERTICALE (EV305) (FM327)

      U     "EV305";
      UN    "BDCV";
      =     DB11.DBX  159.5;
NETWORK
TITLE =SEGN 167 = ATTESA SPINE ROTAZ AVANTI (EV306) (FM322,FM324)

      U     "EV306";
      UN    "SRA";
      =     DB11.DBX  159.6;
NETWORK
TITLE =SEGN 168 = ATTESA SPINE ROTAZ INDIETRO (EV307) (FM323,FM325)

      U     "EV307";
      UN    "SRI";
      =     DB11.DBX  159.7;
NETWORK
TITLE =SEGN 169 = ATTESA TAVOLA RIC ALTA (EV310) (FM332)

      U     "EV310";
      UN    "TRA";
      =     DB11.DBX  158.0;
NETWORK
TITLE =SEGN 170 = ATTESA TAVOLA RIC BASSA (EV311) (FM333)

      U     "EV311";
      UN    "TRB";
      =     DB11.DBX  158.1;
NETWORK
TITLE =SEGN 171 = ATTESA DOSATORE 1 AVANTI (EV312) (FM360)

      U     "EV312";
      UN    "DV1A";
      =     DB11.DBX  158.2;
NETWORK
TITLE =SEGN 172 = ATTESA DOSATORE 1 INDIETRO (EV313) (FM361)

      U     "EV313";
      UN    "DV1I";
      =     DB11.DBX  158.3;
NETWORK
TITLE =SEGN 173 = ATTESA DOSATORE 2 AVANTI (EV314) (FM362)

      U     "EV314";
      UN    "DV2A";
      =     DB11.DBX  158.4;
NETWORK
TITLE =SEGN 174 = ATTESA DOSATORE 2 INDIETRO (EV315) (FM363)

      U     "EV315";
      UN    "DV2I";
      =     DB11.DBX  158.5;
NETWORK
TITLE =SEGN 175 = ATTESA DOSATORE 3 AVANTI (EV316) (FM364)

      U     "EV316";
      UN    "DV3A";
      =     DB11.DBX  158.6;
NETWORK
TITLE =SEGN 176 = ATTESA DOSATORE 3 INDIETRO (EV317) (FM365)
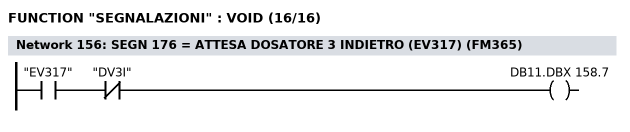
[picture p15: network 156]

      U     "EV317";
      UN    "DV3I";
      =     DB11.DBX  158.7;
NETWORK
TITLE =

// SEGN 177-184 DBB161
// SEGN 185-192 DBB160
// SEGN 193-200 DBB163
// SEGN 201-208 DBB162
// SEGN 209-216 DBB165
// SEGN 217-224 DBB164
// SEGN 225-232 DBB167
// SEGN 233-240 DBB166
// SEGN 241-248 DBB169
// SEGN 249-256 DBB168
END_FUNCTION

